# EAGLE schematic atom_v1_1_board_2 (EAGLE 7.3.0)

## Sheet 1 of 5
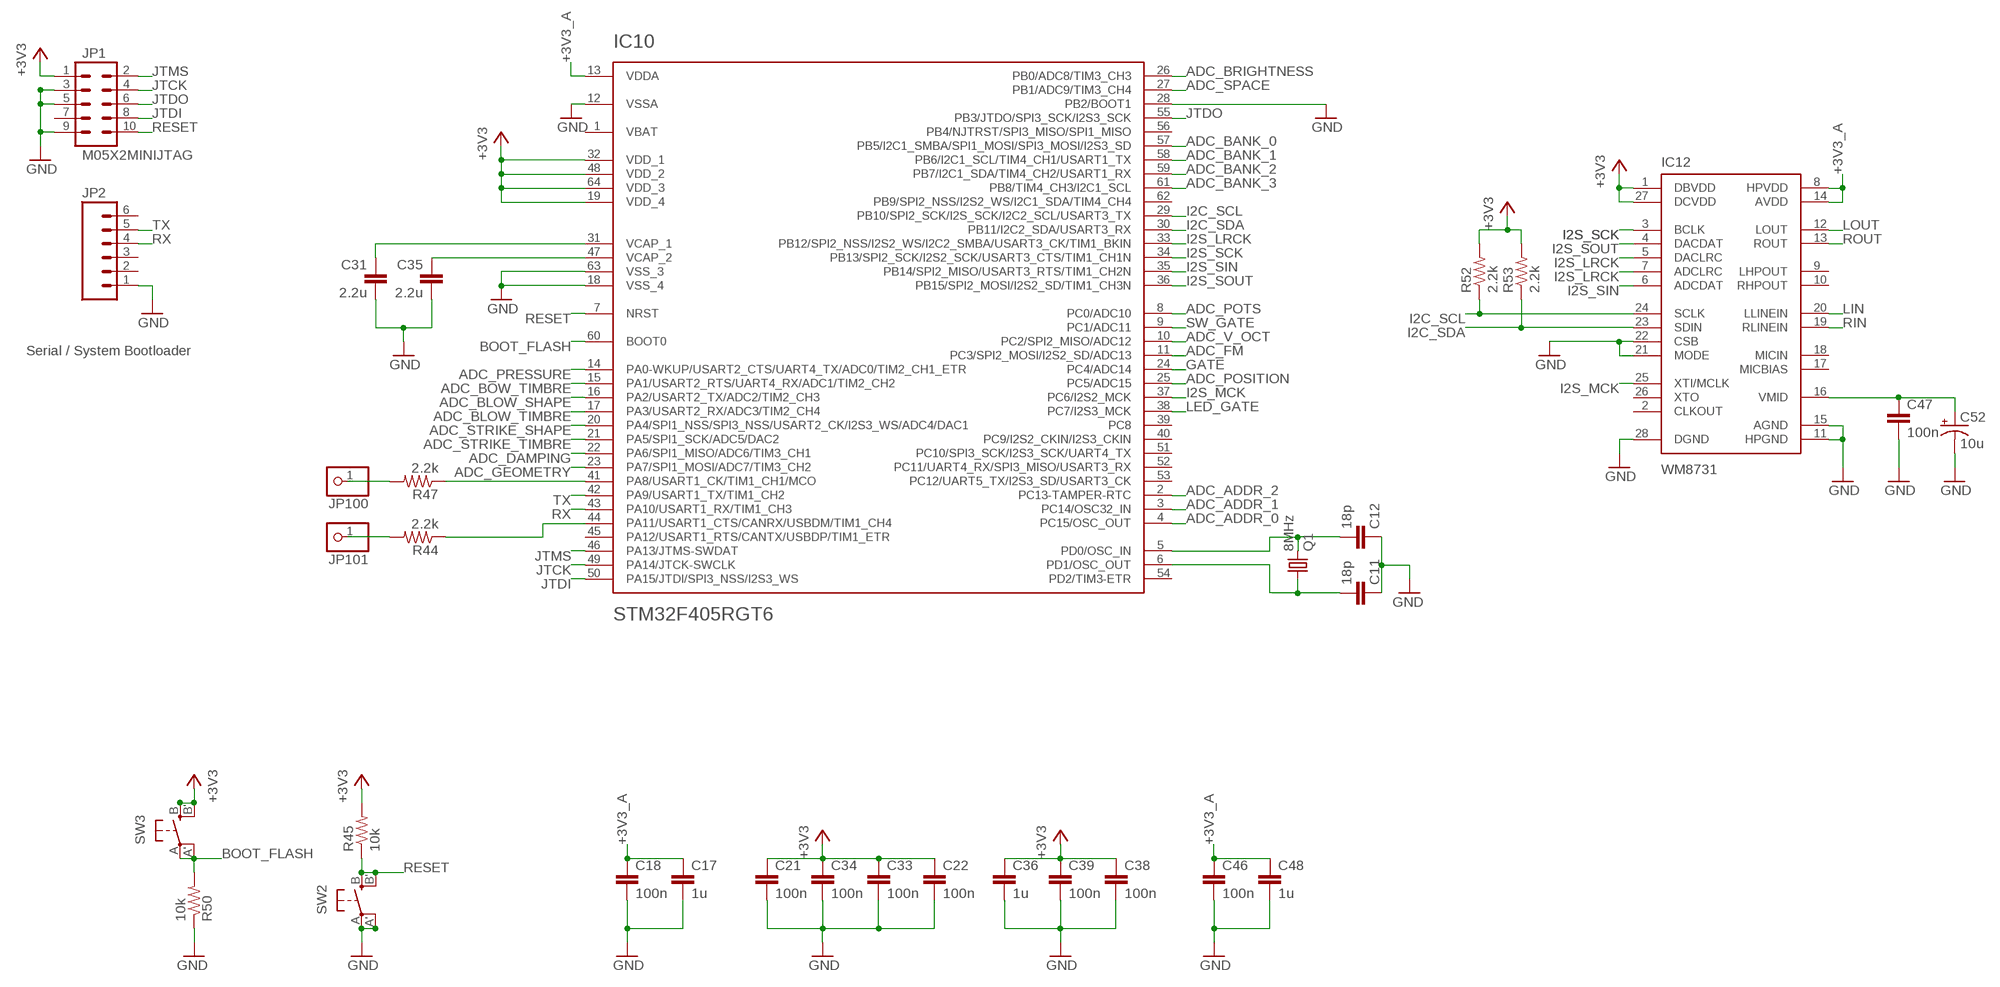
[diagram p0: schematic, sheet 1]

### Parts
C11  18p  CAPACITOR  [RESISTOR_0603]
C12  18p  CAPACITOR  [RESISTOR_0603]
C17  1u  CAPACITOR  [RESISTOR_0603]
C18  100n  CAPACITOR  [RESISTOR_0603]
C21  100n  CAPACITOR  [RESISTOR_0603]
C22  100n  CAPACITOR  [RESISTOR_0603]
C31  2.2u  CAPACITOR  [RESISTOR_0603]
C33  100n  CAPACITOR  [RESISTOR_0603]
C34  100n  CAPACITOR  [RESISTOR_0603]
C35  2.2u  CAPACITOR  [RESISTOR_0603]
C36  1u  CAPACITOR  [RESISTOR_0603]
C38  100n  CAPACITOR  [RESISTOR_0603]
C39  100n  CAPACITOR  [RESISTOR_0603]
C46  100n  CAPACITOR  [RESISTOR_0603]
C47  100n  CAPACITOR  [RESISTOR_0603]
C48  1u  CAPACITOR  [RESISTOR_0603]
C52  10u  CAP_POL  [PANASONIC_B]
IC10  STM32F405RGT6  STM32F20X  [TQFP-10X10-64]
IC12  WM8731  [SSOP28]
JP1  M05X2MINIJTAG  [2X5-1.27]
JP2  M06SIP  [1X06]
JP100  PINHD-1X1  [1X01]
JP101  PINHD-1X1  [1X01]
Q1  8MHz  CRYSTAL  [HC49UP]
R44  2.2k  RESISTOR  [RESISTOR_0603]
R45  10k  RESISTOR  [RESISTOR_0603]
R47  2.2k  RESISTOR  [RESISTOR_0603]
R50  10k  RESISTOR  [RESISTOR_0603]
R52  2.2k  RESISTOR  [RESISTOR_0603]
R53  2.2k  RESISTOR  [RESISTOR_0603]
SW2  EVQQ2  [EVQ-Q2]
SW3  EVQQ2  [EVQ-Q2]

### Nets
+3V3: C21.1 C22.1 C33.1 C34.1 C36.1 C38.1 C39.1 IC10.19(VDD_4) IC10.32(VDD_1) IC10.48(VDD_2) IC10.64(VDD_3) IC12.1(DBVDD) IC12.27(DCVDD) JP1.1 R45.2 R52.2 R53.2 SW3.B'(S1) SW3.B(S) ; also sheet 5
+3V3_A: C17.1 C18.1 C46.1 C48.1 IC10.13(VDDA) IC12.8(HPVDD) IC12.14(AVDD) ; also sheet 3,4,5
ADC_ADDR_0: IC10.4(PC15/OSC_OUT) ; also sheet 4
ADC_ADDR_1: IC10.3(PC14/OSC32_IN) ; also sheet 4
ADC_ADDR_2: IC10.2(PC13-TAMPER-RTC) ; also sheet 4
ADC_BANK_0: IC10.57(PB5/I2C1_SMBA/SPI1_MOSI/SPI3_MOSI/I2S3_SD) ; also sheet 4
ADC_BANK_1: IC10.58(PB6/I2C1_SCL/TIM4_CH1/USART1_TX) ; also sheet 4
ADC_BANK_2: IC10.59(PB7/I2C1_SDA/TIM4_CH2/USART1_RX) ; also sheet 4
ADC_BANK_3: IC10.61(PB8/TIM4_CH3/I2C1_SCL) ; also sheet 4
ADC_BLOW_SHAPE: IC10.16(PA2/USART2_TX/ADC2/TIM2_CH3) ; also sheet 3
ADC_BLOW_TIMBRE: IC10.17(PA3/USART2_RX/ADC3/TIM2_CH4) ; also sheet 3
ADC_BOW_TIMBRE: IC10.15(PA1/USART2_RTS/UART4_RX/ADC1/TIM2_CH2) ; also sheet 3
ADC_BRIGHTNESS: IC10.26(PB0/ADC8/TIM3_CH3) ; also sheet 3
ADC_DAMPING: IC10.22(PA6/SPI1_MISO/ADC6/TIM3_CH1) ; also sheet 3
ADC_FM: IC10.11(PC3/SPI2_MOSI/I2S2_SD/ADC13) ; also sheet 3
ADC_GEOMETRY: IC10.23(PA7/SPI1_MOSI/ADC7/TIM3_CH2) ; also sheet 3
ADC_POSITION: IC10.25(PC5/ADC15) ; also sheet 3
ADC_POTS: IC10.8(PC0/ADC10) ; also sheet 4
ADC_PRESSURE: IC10.14(PA0-WKUP/USART2_CTS/UART4_TX/ADC0/TIM2_CH1_ETR) ; also sheet 3
ADC_SPACE: IC10.27(PB1/ADC9/TIM3_CH4) ; also sheet 3
ADC_STRIKE_SHAPE: IC10.20(PA4/SPI1_NSS/SPI3_NSS/USART2_CK/I2S3_WS/ADC4/DAC1) ; also sheet 3
ADC_STRIKE_TIMBRE: IC10.21(PA5/SPI1_SCK/ADC5/DAC2) ; also sheet 3
ADC_V_OCT: IC10.10(PC2/SPI2_MISO/ADC12) ; also sheet 3
BOOT_FLASH: IC10.60(BOOT0) R50.2 SW3.A'(P1) SW3.A(P)
GATE: IC10.24(PC4/ADC14) ; also sheet 4
GND: C11.1 C12.1 C17.2 C18.2 C21.2 C22.2 C31.2 C33.2 C34.2 C35.2 C36.2 C38.2 C39.2 C46.2 C47.2 C48.2 C52.- IC10.12(VSSA) IC10.18(VSS_4) IC10.28(PB2/BOOT1) IC10.63(VSS_3) IC12.11(HPGND) IC12.15(AGND) IC12.21(MODE) IC12.22(CSB) IC12.28(DGND) JP1.3 JP1.5 JP1.9 JP2.1 R50.1 SW2.A'(P1) SW2.A(P) ; also sheet 2,3,4,5
I2C_SCL: IC10.29(PB10/SPI2_SCK/I2S_SCK/I2C2_SCL/USART3_TX) IC12.24(SCLK) R52.1
I2C_SDA: IC10.30(PB11/I2C2_SDA/USART3_RX) IC12.23(SDIN) R53.1
I2S_LRCK: IC10.33(PB12/SPI2_NSS/I2S2_WS/I2C2_SMBA/USART3_CK/TIM1_BKIN) IC12.5(DACLRC) IC12.7(ADCLRC)
I2S_MCK: IC10.37(PC6/I2S2_MCK) IC12.25(XTI/MCLK)
I2S_SCK: IC10.34(PB13/SPI2_SCK/I2S2_SCK/USART3_CTS/TIM1_CH1N) IC12.3(BCLK)
I2S_SIN: IC10.35(PB14/SPI2_MISO/USART3_RTS/TIM1_CH2N) IC12.6(ADCDAT)
I2S_SOUT: IC10.36(PB15/SPI2_MOSI/I2S2_SD/TIM1_CH3N) IC12.4(DACDAT)
JTCK: IC10.49(PA14/JTCK-SWCLK) JP1.4
JTDI: IC10.50(PA15/JTDI/SPI3_NSS/I2S3_WS) JP1.8
JTDO: IC10.55(PB3/JTDO/SPI3_SCK/I2S3_SCK) JP1.6
JTMS: IC10.46(PA13/JTMS-SWDAT) JP1.2
LED_GATE: IC10.38(PC7/I2S3_MCK) ; also sheet 4
LIN: IC12.20(LLINEIN) ; also sheet 2
LOUT: IC12.12(LOUT) ; also sheet 2
N$7: C12.2 IC10.5(PD0/OSC_IN) Q1.2
N$8: C11.2 IC10.6(PD1/OSC_OUT) Q1.1
N$13: C35.1 IC10.47(VCAP_2)
N$17: C47.1 C52.+ IC12.16(VMID)
N$19: C31.1 IC10.31(VCAP_1)
N$54: IC10.44(PA11/USART1_CTS/CANRX/USBDM/TIM1_CH4) R44.1
N$79: IC10.41(PA8/USART1_CK/TIM1_CH1/MCO) R47.1
N$129: JP100.1 R47.2
N$130: JP101.1 R44.2
RESET: IC10.7(NRST) JP1.10 R45.1 SW2.B'(S1) SW2.B(S)
RIN: IC12.19(RLINEIN) ; also sheet 2
ROUT: IC12.13(ROUT) ; also sheet 2
RX: IC10.43(PA10/USART1_RX/TIM1_CH3) JP2.4
SW_GATE: IC10.9(PC1/ADC11) ; also sheet 4
TX: IC10.42(PA9/USART1_TX/TIM1_CH2) JP2.5
Unconnected: IC10.39(PC8) IC10.40(PC9/I2S2_CKIN/I2S3_CKIN) IC10.45(PA12/USART1_RTS/CANTX/USBDP/TIM1_ETR) IC10.51(PC10/SPI3_SCK/I2S3_SCK/UART4_TX) IC10.52(PC11/UART4_RX/SPI3_MISO/USART3_RX) IC10.53(PC12/UART5_TX/I2S3_SD/USART3_CK) IC10.54(PD2/TIM3-ETR) IC10.56(PB4/NJTRST/SPI3_MISO/SPI1_MISO) IC10.62(PB9/SPI2_NSS/I2S2_WS/I2C1_SDA/TIM4_CH4) IC12.2(CLKOUT) IC12.9(LHPOUT) IC12.10(RHPOUT) IC12.17(MICBIAS) IC12.18(MICIN) IC12.26(XTO) JP1.7 JP2.2 JP2.3 JP2.6

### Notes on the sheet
- Serial / System Bootloader

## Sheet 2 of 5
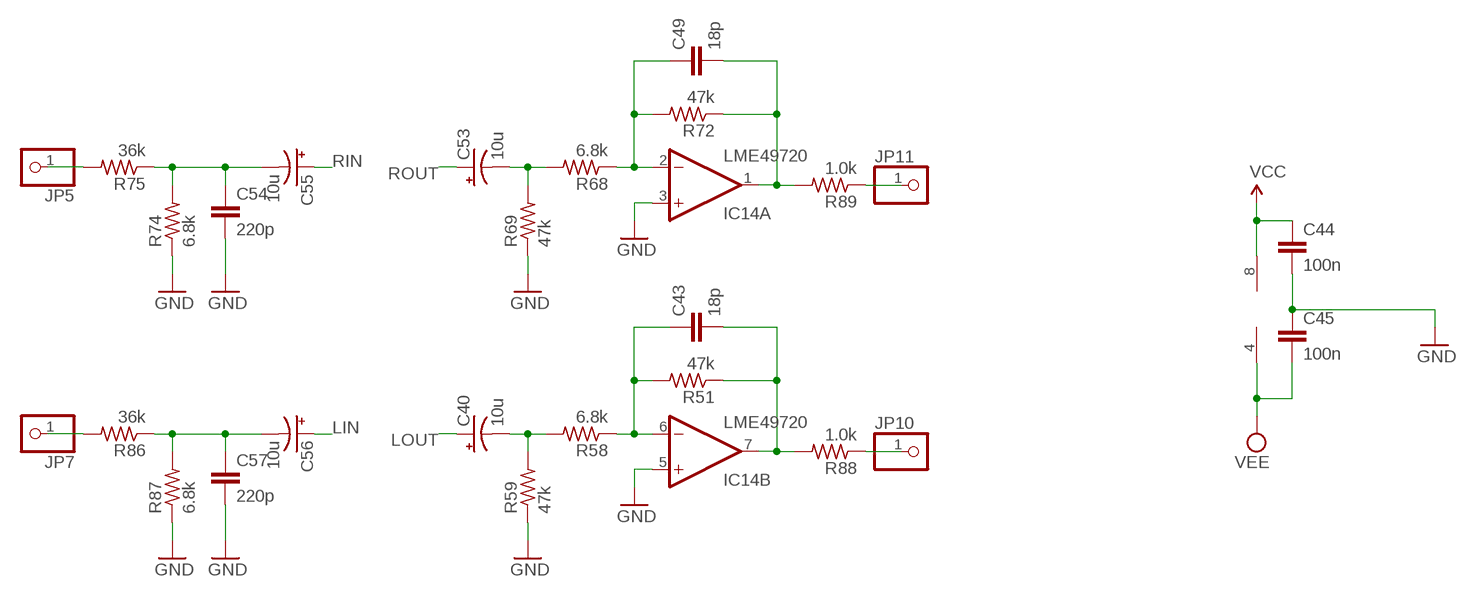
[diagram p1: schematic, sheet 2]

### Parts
C40  10u  CAP_POL  [PANASONIC_B]
C43  18p  CAPACITOR  [RESISTOR_0603]
C44  100n  CAPACITOR  [RESISTOR_0603]
C45  100n  CAPACITOR  [RESISTOR_0603]
C49  18p  CAPACITOR  [RESISTOR_0603]
C53  10u  CAP_POL  [PANASONIC_B]
C54  220p  CAPACITOR  [RESISTOR_0603]
C55  10u  CAP_POL  [PANASONIC_B]
C56  10u  CAP_POL  [PANASONIC_B]
C57  220p  CAPACITOR  [RESISTOR_0603]
IC14  LME49720  TL072D  [SO08]
JP5  PINHD-1X1  [1X01]
JP7  PINHD-1X1  [1X01]
JP10  PINHD-1X1  [1X01]
JP11  PINHD-1X1  [1X01]
R51  47k  RESISTOR  [RESISTOR_0603]
R58  6.8k  RESISTOR  [RESISTOR_0603]
R59  47k  RESISTOR  [RESISTOR_0603]
R68  6.8k  RESISTOR  [RESISTOR_0603]
R69  47k  RESISTOR  [RESISTOR_0603]
R72  47k  RESISTOR  [RESISTOR_0603]
R74  6.8k  RESISTOR  [RESISTOR_0603]
R75  36k  RESISTOR  [RESISTOR_0603]
R86  36k  RESISTOR  [RESISTOR_0603]
R87  6.8k  RESISTOR  [RESISTOR_0603]
R88  1.0k  RESISTOR  [RESISTOR_0603]
R89  1.0k  RESISTOR  [RESISTOR_0603]

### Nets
GND: C44.2 C45.1 C54.2 C57.2 IC14.3(A:+IN) IC14.5(B:+IN) R59.1 R69.1 R74.1 R87.1 ; also sheet 1,3,4,5
LIN: C56.+ ; also sheet 1
LOUT: C40.+ ; also sheet 1
N$18: C56.- C57.1 R86.1 R87.2
N$22: C54.1 C55.- R74.2 R75.1
N$23: C40.- R58.2 R59.2
N$25: C43.1 IC14.6(B:-IN) R51.2 R58.1
N$28: C43.2 IC14.7(B:OUT) R51.1 R88.2
N$31: C53.- R68.2 R69.2
N$32: C49.1 IC14.2(A:-IN) R68.1 R72.2
N$33: C49.2 IC14.1(A:OUT) R72.1 R89.2
N$81: JP5.1 R75.2
N$82: JP11.1 R89.1
N$84: JP10.1 R88.1
N$86: JP7.1 R86.2
RIN: C55.+ ; also sheet 1
ROUT: C53.+ ; also sheet 1
VCC [wide]: C44.1 IC14.8(P:V+) ; also sheet 5
VEE [wide]: C45.2 IC14.4(P:V-) ; also sheet 5

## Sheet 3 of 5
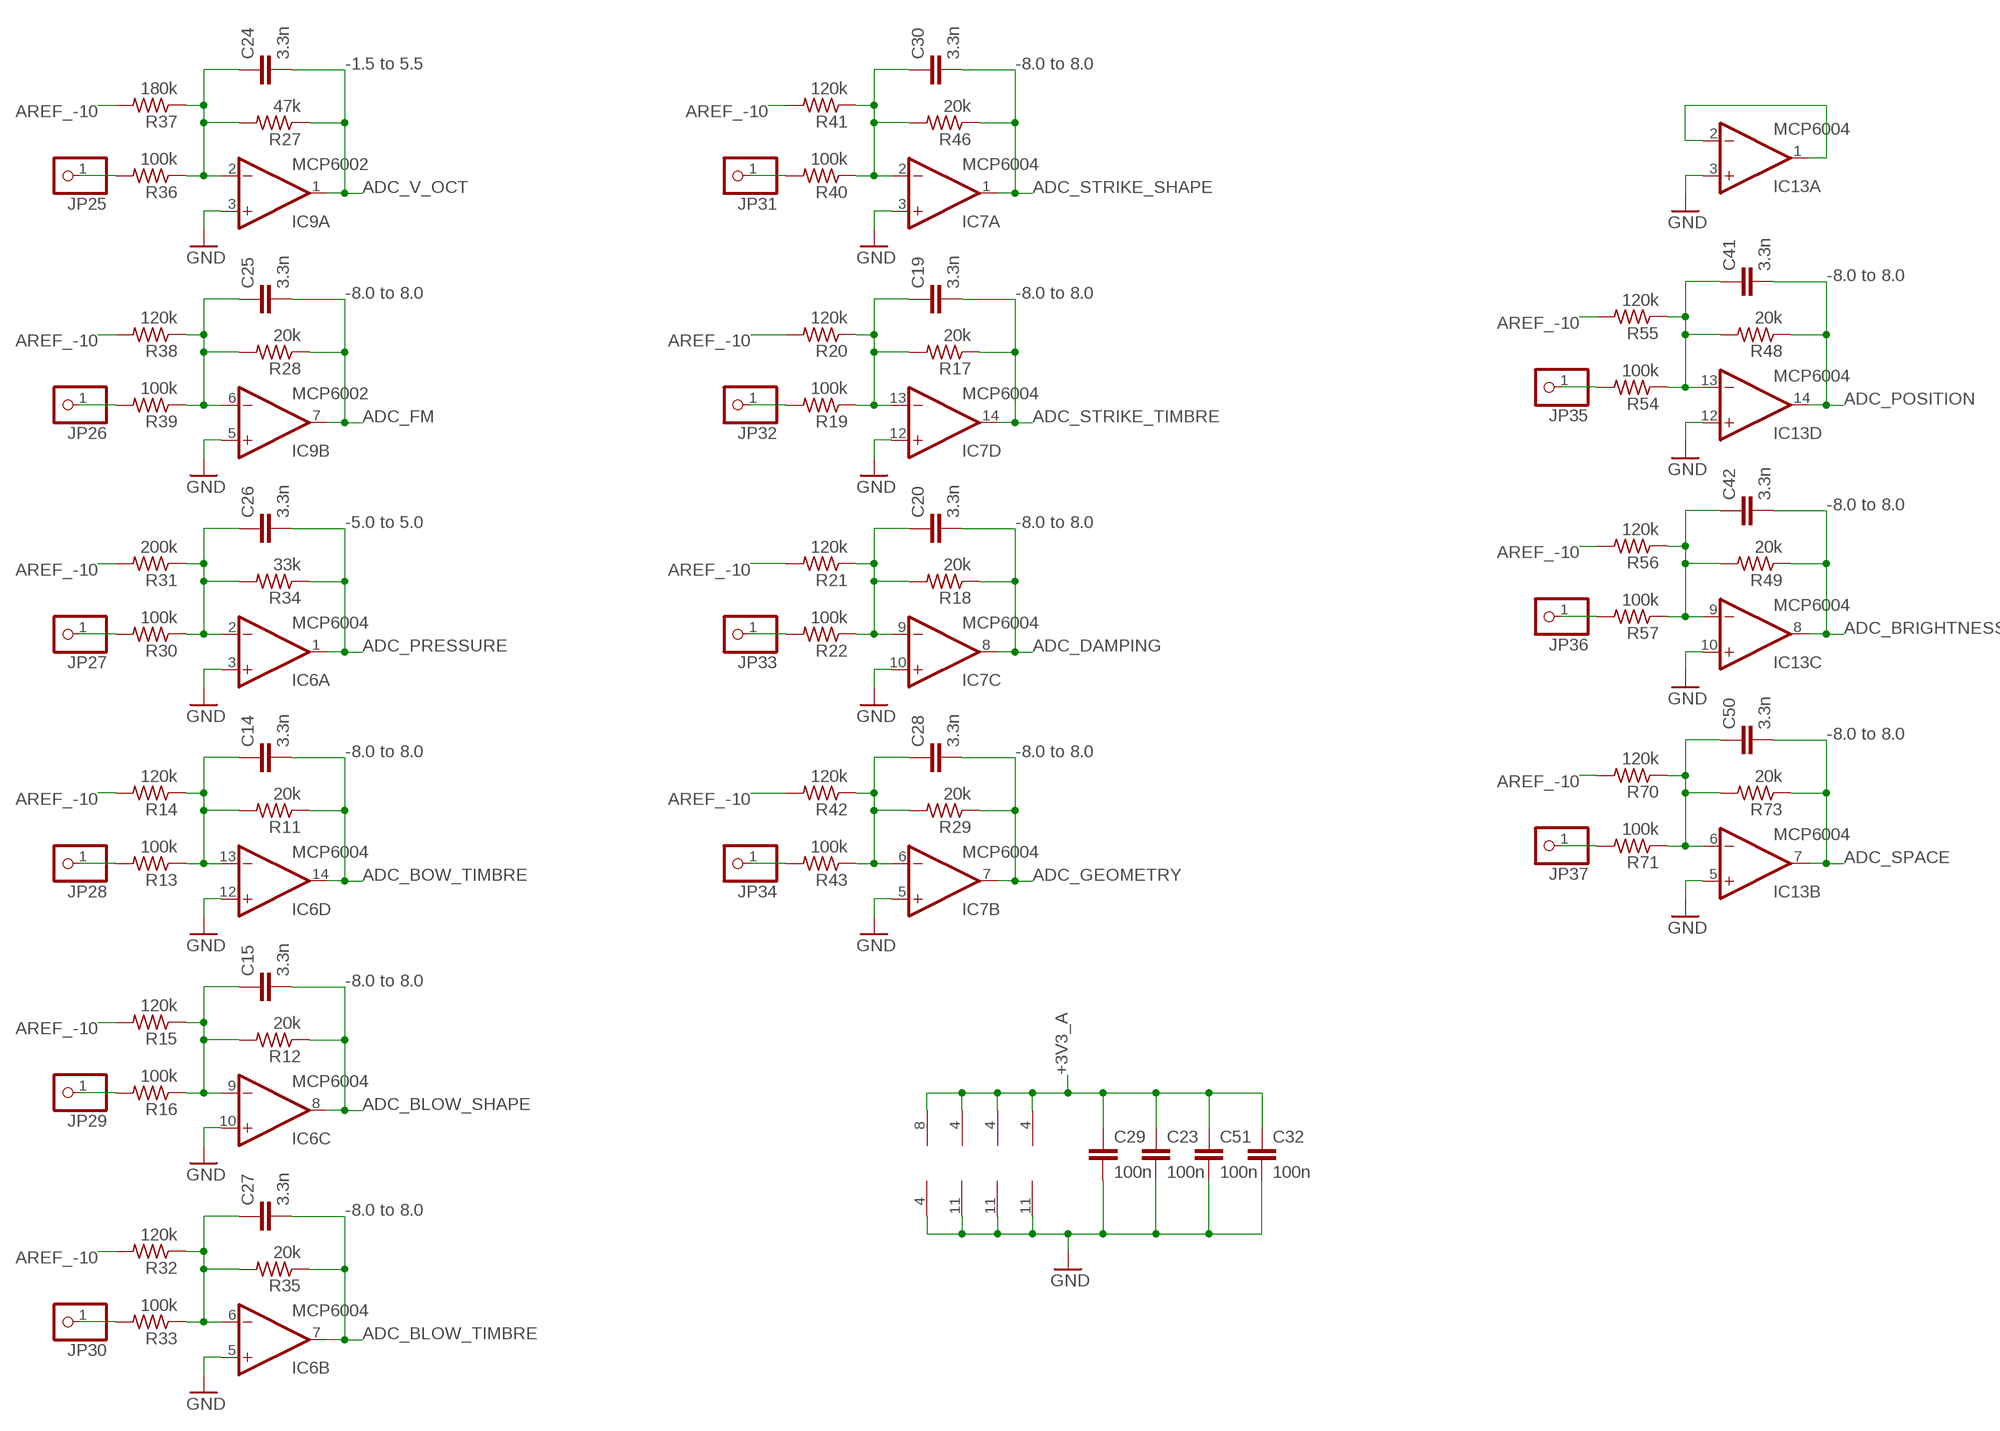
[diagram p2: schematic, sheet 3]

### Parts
C14  3.3n  CAPACITOR  [RESISTOR_0603]
C15  3.3n  CAPACITOR  [RESISTOR_0603]
C19  3.3n  CAPACITOR  [RESISTOR_0603]
C20  3.3n  CAPACITOR  [RESISTOR_0603]
C23  100n  CAPACITOR  [RESISTOR_0603]
C24  3.3n  CAPACITOR  [RESISTOR_0603]
C25  3.3n  CAPACITOR  [RESISTOR_0603]
C26  3.3n  CAPACITOR  [RESISTOR_0603]
C27  3.3n  CAPACITOR  [RESISTOR_0603]
C28  3.3n  CAPACITOR  [RESISTOR_0603]
C29  100n  CAPACITOR  [RESISTOR_0603]
C30  3.3n  CAPACITOR  [RESISTOR_0603]
C32  100n  CAPACITOR  [RESISTOR_0603]
C41  3.3n  CAPACITOR  [RESISTOR_0603]
C42  3.3n  CAPACITOR  [RESISTOR_0603]
C50  3.3n  CAPACITOR  [RESISTOR_0603]
C51  100n  CAPACITOR  [RESISTOR_0603]
IC6  MCP6004  TL074D  [SO14]
IC7  MCP6004  TL074D  [SO14]
IC9  MCP6002  TL072D  [SO08]
IC13  MCP6004  TL074D  [SO14]
JP25  PINHD-1X1  [1X01]
JP26  PINHD-1X1  [1X01]
JP27  PINHD-1X1  [1X01]
JP28  PINHD-1X1  [1X01]
JP29  PINHD-1X1  [1X01]
JP30  PINHD-1X1  [1X01]
JP31  PINHD-1X1  [1X01]
JP32  PINHD-1X1  [1X01]
JP33  PINHD-1X1  [1X01]
JP34  PINHD-1X1  [1X01]
JP35  PINHD-1X1  [1X01]
JP36  PINHD-1X1  [1X01]
JP37  PINHD-1X1  [1X01]
R11  20k  RESISTOR  [RESISTOR_0603]
R12  20k  RESISTOR  [RESISTOR_0603]
R13  100k  RESISTOR  [RESISTOR_0603]
R14  120k  RESISTOR  [RESISTOR_0603]
R15  120k  RESISTOR  [RESISTOR_0603]
R16  100k  RESISTOR  [RESISTOR_0603]
R17  20k  RESISTOR  [RESISTOR_0603]
R18  20k  RESISTOR  [RESISTOR_0603]
R19  100k  RESISTOR  [RESISTOR_0603]
R20  120k  RESISTOR  [RESISTOR_0603]
R21  120k  RESISTOR  [RESISTOR_0603]
R22  100k  RESISTOR  [RESISTOR_0603]
R27  47k  RESISTOR  [RESISTOR_0603]
R28  20k  RESISTOR  [RESISTOR_0603]
R29  20k  RESISTOR  [RESISTOR_0603]
R30  100k  RESISTOR  [RESISTOR_0603]
R31  200k  RESISTOR  [RESISTOR_0603]
R32  120k  RESISTOR  [RESISTOR_0603]
R33  100k  RESISTOR  [RESISTOR_0603]
R34  33k  RESISTOR  [RESISTOR_0603]
R35  20k  RESISTOR  [RESISTOR_0603]
R36  100k  RESISTOR  [RESISTOR_0603]
R37  180k  RESISTOR  [RESISTOR_0603]
R38  120k  RESISTOR  [RESISTOR_0603]
R39  100k  RESISTOR  [RESISTOR_0603]
R40  100k  RESISTOR  [RESISTOR_0603]
R41  120k  RESISTOR  [RESISTOR_0603]
R42  120k  RESISTOR  [RESISTOR_0603]
R43  100k  RESISTOR  [RESISTOR_0603]
R46  20k  RESISTOR  [RESISTOR_0603]
R48  20k  RESISTOR  [RESISTOR_0603]
R49  20k  RESISTOR  [RESISTOR_0603]
R54  100k  RESISTOR  [RESISTOR_0603]
R55  120k  RESISTOR  [RESISTOR_0603]
R56  120k  RESISTOR  [RESISTOR_0603]
R57  100k  RESISTOR  [RESISTOR_0603]
R70  120k  RESISTOR  [RESISTOR_0603]
R71  100k  RESISTOR  [RESISTOR_0603]
R73  20k  RESISTOR  [RESISTOR_0603]

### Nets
+3V3_A: C23.1 C29.1 C32.1 C51.1 IC6.4(P:V+) IC7.4(P:V+) IC9.8(P:V+) IC13.4(P:V+) ; also sheet 1,4,5
ADC_BLOW_SHAPE: C15.2 IC6.8(C:OUT) R12.1 ; also sheet 1
ADC_BLOW_TIMBRE: C27.2 IC6.7(B:OUT) R35.1 ; also sheet 1
ADC_BOW_TIMBRE: C14.2 IC6.14(D:OUT) R11.1 ; also sheet 1
ADC_BRIGHTNESS: C42.2 IC13.8(C:OUT) R49.1 ; also sheet 1
ADC_DAMPING: C20.2 IC7.8(C:OUT) R18.1 ; also sheet 1
ADC_FM: C25.2 IC9.7(B:OUT) R28.1 ; also sheet 1
ADC_GEOMETRY: C28.2 IC7.7(B:OUT) R29.1 ; also sheet 1
ADC_POSITION: C41.2 IC13.14(D:OUT) R48.1 ; also sheet 1
ADC_PRESSURE: C26.2 IC6.1(A:OUT) R34.1 ; also sheet 1
ADC_SPACE: C50.2 IC13.7(B:OUT) R73.1 ; also sheet 1
ADC_STRIKE_SHAPE: C30.2 IC7.1(A:OUT) R46.1 ; also sheet 1
ADC_STRIKE_TIMBRE: C19.2 IC7.14(D:OUT) R17.1 ; also sheet 1
ADC_V_OCT: C24.2 IC9.1(A:OUT) R27.1 ; also sheet 1
AREF_-10: R14.2 R15.2 R20.2 R21.2 R31.2 R32.2 R37.2 R38.2 R41.2 R42.2 R55.2 R56.2 R70.2 ; also sheet 5
GND: C23.2 C29.2 C32.2 C51.2 IC6.3(A:+IN) IC6.5(B:+IN) IC6.10(C:+IN) IC6.11(P:V-) IC6.12(D:+IN) IC7.3(A:+IN) IC7.5(B:+IN) IC7.10(C:+IN) IC7.11(P:V-) IC7.12(D:+IN) IC9.3(A:+IN) IC9.4(P:V-) IC9.5(B:+IN) IC13.3(A:+IN) IC13.5(B:+IN) IC13.10(C:+IN) IC13.11(P:V-) IC13.12(D:+IN) ; also sheet 1,2,4,5
N$2: C15.1 IC6.9(C:-IN) R12.2 R15.1 R16.1
N$4: JP25.1 R36.2
N$5: C14.1 IC6.13(D:-IN) R11.2 R13.1 R14.1
N$9: C19.1 IC7.13(D:-IN) R17.2 R19.1 R20.1
N$10: JP26.1 R39.2
N$11: C24.1 IC9.2(A:-IN) R27.2 R36.1 R37.1
N$14: C20.1 IC7.9(C:-IN) R18.2 R21.1 R22.1
N$15: C25.1 IC9.6(B:-IN) R28.2 R38.1 R39.1
N$24: C30.1 IC7.2(A:-IN) R40.1 R41.1 R46.2
N$27: C27.1 IC6.6(B:-IN) R32.1 R33.1 R35.2
N$30: C42.1 IC13.9(C:-IN) R49.2 R56.1 R57.1
N$35: C50.1 IC13.6(B:-IN) R70.1 R71.1 R73.2
N$37: C28.1 IC7.6(B:-IN) R29.2 R42.1 R43.1
N$40: C41.1 IC13.13(D:-IN) R48.2 R54.1 R55.1
N$41: JP27.1 R30.2
N$42: C26.1 IC6.2(A:-IN) R30.1 R31.1 R34.2
N$44: IC13.1(A:OUT) IC13.2(A:-IN)
N$87: JP28.1 R13.2
N$88: JP29.1 R16.2
N$89: JP30.1 R33.2
N$93: JP31.1 R40.2
N$94: JP32.1 R19.2
N$95: JP33.1 R22.2
N$96: JP34.1 R43.2
N$97: JP37.1 R71.2
N$98: JP36.1 R57.2
N$99: JP35.1 R54.2

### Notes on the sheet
- -1.5 to 5.5 | -8.0 to 8.0
- -8.0 to 8.0
- -8.0 to 8.0 | -8.0 to 8.0
- -8.0 to 8.0
- -5.0 to 5.0 | -8.0 to 8.0
- -8.0 to 8.0
- -8.0 to 8.0 | -8.0 to 8.0
- -8.0 to 8.0
- -8.0 to 8.0

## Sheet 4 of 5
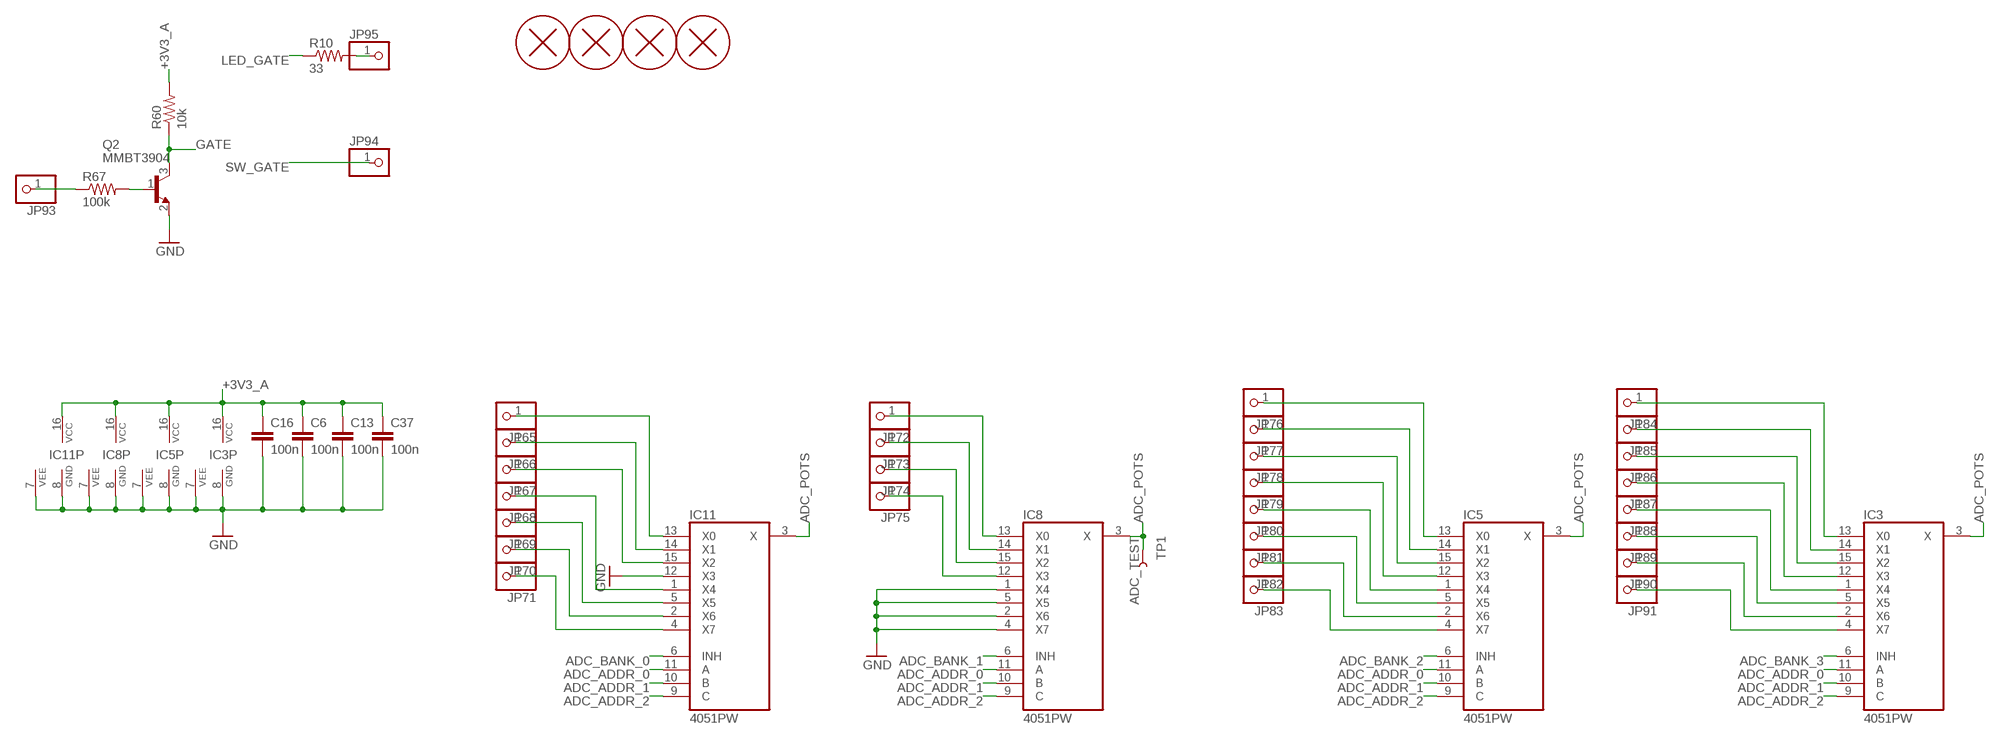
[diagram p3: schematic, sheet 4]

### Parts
C6  100n  CAPACITOR  [RESISTOR_0603]
C13  100n  CAPACITOR  [RESISTOR_0603]
C16  100n  CAPACITOR  [RESISTOR_0603]
C37  100n  CAPACITOR  [RESISTOR_0603]
H1  PCB_SCREW  [PCB_SCREW]
H2  PCB_SCREW  [PCB_SCREW]
H3  PCB_SCREW  [PCB_SCREW]
H4  PCB_SCREW  [PCB_SCREW]
IC3  4051PW  [TSSOP16]
IC5  4051PW  [TSSOP16]
IC8  4051PW  [TSSOP16]
IC11  4051PW  [TSSOP16]
JP65  PINHD-1X1  [1X01]
JP66  PINHD-1X1  [1X01]
JP67  PINHD-1X1  [1X01]
JP68  PINHD-1X1  [1X01]
JP69  PINHD-1X1  [1X01]
JP70  PINHD-1X1  [1X01]
JP71  PINHD-1X1  [1X01]
JP72  PINHD-1X1  [1X01]
JP73  PINHD-1X1  [1X01]
JP74  PINHD-1X1  [1X01]
JP75  PINHD-1X1  [1X01]
JP76  PINHD-1X1  [1X01]
JP77  PINHD-1X1  [1X01]
JP78  PINHD-1X1  [1X01]
JP79  PINHD-1X1  [1X01]
JP80  PINHD-1X1  [1X01]
JP81  PINHD-1X1  [1X01]
JP82  PINHD-1X1  [1X01]
JP83  PINHD-1X1  [1X01]
JP84  PINHD-1X1  [1X01]
JP85  PINHD-1X1  [1X01]
JP86  PINHD-1X1  [1X01]
JP87  PINHD-1X1  [1X01]
JP88  PINHD-1X1  [1X01]
JP89  PINHD-1X1  [1X01]
JP90  PINHD-1X1  [1X01]
JP91  PINHD-1X1  [1X01]
JP93  PINHD-1X1  [1X01]
JP94  PINHD-1X1  [1X01]
JP95  PINHD-1X1  [1X01]
Q2  MMBT3904  MMBT3904SOT23  [SOT23]
R10  33  RESISTOR  [RESISTOR_0603]
R60  10k  RESISTOR  [RESISTOR_0603]
R67  100k  RESISTOR  [RESISTOR_0603]
TP1  ADC_TEST  TEST-POINT3  [PAD.03X.03]

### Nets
+3V3_A: C6.1 C13.1 C16.1 C37.1 IC3.16(VCC) IC5.16(VCC) IC8.16(VCC) IC11.16(VCC) R60.2 ; also sheet 1,3,5
ADC_ADDR_0: IC3.11(A) IC5.11(A) IC8.11(A) IC11.11(A) ; also sheet 1
ADC_ADDR_1: IC3.10(B) IC5.10(B) IC8.10(B) IC11.10(B) ; also sheet 1
ADC_ADDR_2: IC3.9(C) IC5.9(C) IC8.9(C) IC11.9(C) ; also sheet 1
ADC_BANK_0: IC11.6(INH) ; also sheet 1
ADC_BANK_1: IC8.6(INH) ; also sheet 1
ADC_BANK_2: IC5.6(INH) ; also sheet 1
ADC_BANK_3: IC3.6(INH) ; also sheet 1
ADC_POTS: IC3.3(X) IC5.3(X) IC8.3(X) IC11.3(X) TP1.P$1 ; also sheet 1
GATE: Q2.3(C) R60.1 ; also sheet 1
GND: C6.2 C13.2 C16.2 C37.2 IC3.7(VEE) IC3.8(GND) IC5.7(VEE) IC5.8(GND) IC8.1(X4) IC8.2(X6) IC8.4(X7) IC8.5(X5) IC8.7(VEE) IC8.8(GND) IC11.7(VEE) IC11.8(GND) IC11.12(X3) Q2.2(E) ; also sheet 1,2,3,5
LED_GATE: R10.1 ; also sheet 1
N$38: JP95.1 R10.2
N$66: Q2.1(B) R67.2
N$100: IC11.13(X0) JP65.1
N$101: IC11.14(X1) JP66.1
N$102: IC11.15(X2) JP67.1
N$103: IC11.1(X4) JP68.1
N$104: IC11.5(X5) JP69.1
N$105: IC11.2(X6) JP70.1
N$106: IC11.4(X7) JP71.1
N$107: IC8.13(X0) JP72.1
N$108: IC8.14(X1) JP73.1
N$109: IC8.15(X2) JP74.1
N$110: IC8.12(X3) JP75.1
N$111: IC5.13(X0) JP76.1
N$112: IC5.14(X1) JP77.1
N$113: IC5.15(X2) JP78.1
N$114: IC5.12(X3) JP79.1
N$115: IC5.1(X4) JP80.1
N$116: IC5.5(X5) JP81.1
N$117: IC5.2(X6) JP82.1
N$118: IC5.4(X7) JP83.1
N$119: IC3.13(X0) JP84.1
N$120: IC3.14(X1) JP85.1
N$121: IC3.15(X2) JP86.1
N$122: IC3.12(X3) JP87.1
N$123: IC3.1(X4) JP88.1
N$124: IC3.5(X5) JP89.1
N$125: IC3.2(X6) JP90.1
N$126: IC3.4(X7) JP91.1
N$127: JP93.1 R67.1
SW_GATE: JP94.1 ; also sheet 1

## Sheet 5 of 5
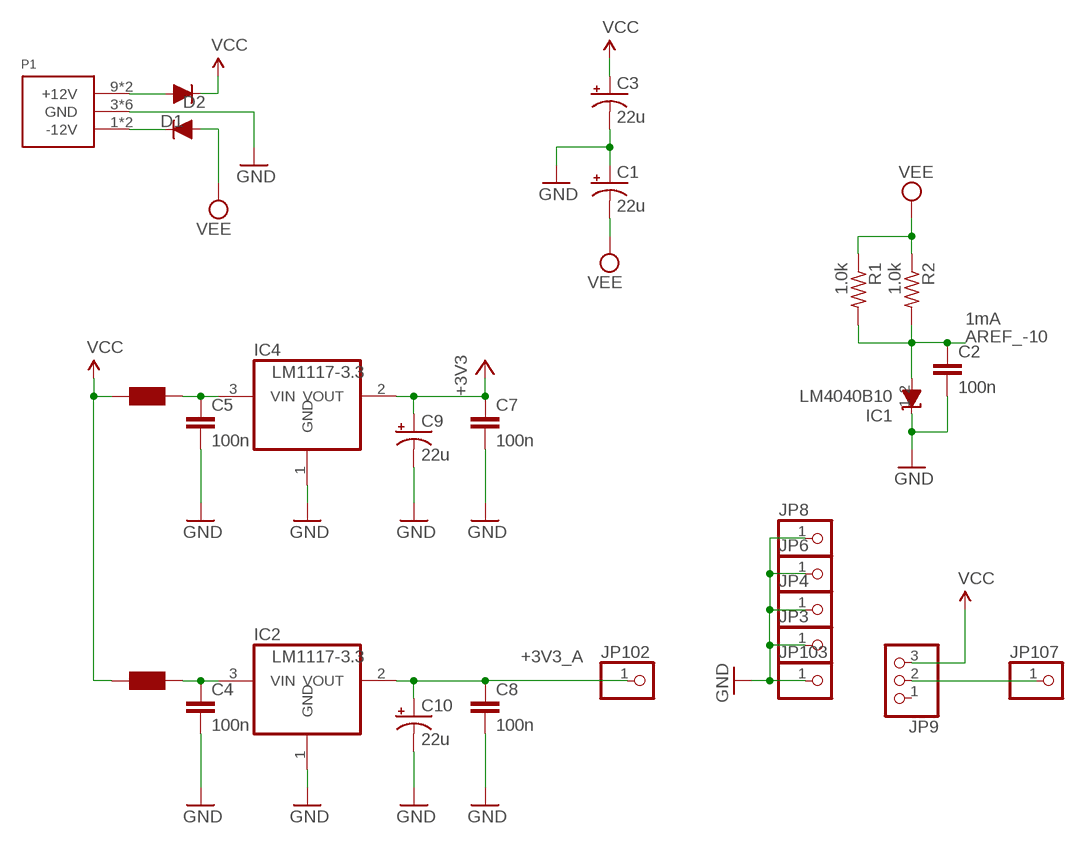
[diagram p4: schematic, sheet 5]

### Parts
C1  22u  CAP_POLD  [PANASONIC_D]
C2  100n  CAPACITOR  [RESISTOR_0603]
C3  22u  CAP_POLD  [PANASONIC_D]
C4  100n  CAPACITOR  [RESISTOR_0603]
C5  100n  CAPACITOR  [RESISTOR_0603]
C7  100n  CAPACITOR  [RESISTOR_0603]
C8  100n  CAPACITOR  [RESISTOR_0603]
C9  22u  CAP_POLD  [PANASONIC_D]
C10  22u  CAP_POLD  [PANASONIC_D]
D1  1N5819HW  DIODE  [SOD123]
D2  1N5819HW  DIODE  [SOD123]
F1  FERRITE-BEAD  [RESISTOR_0603]
F2  FERRITE-BEAD  [RESISTOR_0603]
IC1  LM4040B10  LM4040SOT23  [SOT23]
IC2  LM1117-3.3  REG1117  [SOT223]
IC4  LM1117-3.3  REG1117  [SOT223]
JP3  PINHD-1X1  [1X01]
JP4  PINHD-1X1  [1X01]
JP6  PINHD-1X1  [1X01]
JP8  PINHD-1X1  [1X01]
JP9  PINHD-1X3  [1X03]
JP102  PINHD-1X1  [1X01]
JP103  PINHD-1X1  [1X01]
JP107  PINHD-1X1  [1X01]
P1  POWER_SIMPLE10  [POWER_10]
R1  1.0k  RESISTOR  [RESISTOR_0603]
R2  1.0k  RESISTOR  [RESISTOR_0603]

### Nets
+3V3: C7.1 C9.+ IC4.2(VOUT) ; also sheet 1
+3V3_A: C8.1 C10.+ IC2.2(VOUT) JP102.1 ; also sheet 1,3,4
AREF_-10: C2.1 IC1.2(A) R1.2 R2.2 ; also sheet 3
GND: C1.+ C2.2 C3.- C4.2 C5.2 C7.2 C8.2 C9.- C10.- IC1.1(C) IC2.1(GND) IC4.1(GND) JP3.1 JP4.1 JP6.1 JP8.1 JP103.1 P1.3(GND) P1.4(GND) P1.5(GND) P1.6(GND) P1.7(GND) P1.8(GND) ; also sheet 1,2,3,4
N$1 [wide]: D1.+ P1.9(+12V) P1.10(+12V)
N$3 [wide]: D2.- P1.1(-12V) P1.2(-12V)
N$6 [wide]: JP9.2 JP107.1
N$61 [wide]: C5.1 F1.1 IC4.3(VIN)
N$80 [wide]: C4.1 F2.1 IC2.3(VIN)
VCC [wide]: C3.+ D1.- F1.2 F2.2 JP9.3 ; also sheet 2
VEE [wide]: C1.- D2.+ R1.1 R2.1 ; also sheet 2
Unconnected: JP9.1

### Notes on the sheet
- 1mA

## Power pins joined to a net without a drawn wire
VBAT: IC10.1(VBAT)

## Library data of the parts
C1 C3 C9 C10 C40 C52 C53 C55 C56 = parts_aman:CAP_POL
C2 C4-C8 C11-C39 C41-C51 C54 C57 = parts_aman:CAPACITOR
D1 D2 = parts_aman:DIODE
F1 F2 = parts_aman:FERRITE-BEAD
H1-H4 = parts_aman:PCB_SCREW
IC1 = parts_aman:LM4040
IC2 IC4 = og-vreg:REG1117: 800mA and 1A Low Dropout (LDO) Positive Regulator 1.8V, 2.5V, 2.85V, 3.3V, 5V, and Adj
IC3 IC5 IC8 IC11 = og-ics:4051: 8-channel ANALOG MULTIPLEXER
IC6 IC7 IC13 = gm-ics:TL074: OP AMP
IC9 = gm-ics:TL072: OP AMP
IC10 = og-stm32f2:STM32F20X
IC12 = og-dac:WM8731
IC14 = og-linear:TL072: OP AMP
JP1 = og-header:M05X2: Header 5x2 Standard 10-pin dual row 0.1" header. Commonly used with AVR-ISP. Use with Spark Fun Electronics SKU: PRT-00778
JP2 = SparkFun:M06: Header 6 Standard 6-pin 0.1" header. Use with straight break away headers (SKU : PRT-00116), right angle break away headers (PRT-00553), swiss pins (PRT-00743), machine pins (PRT-00117), and female headers (PRT-00115). Molex polarized connector foot print use with SKU : PRT-08094 with associated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
JP3-JP8 JP10 JP11 JP25-JP37 JP65-JP91 JP93-JP95 JP100-JP103 JP107 = parts_aman:PINHD-1X1: PIN HEADER
JP9 = parts_aman:PINHD-1X3: PIN HEADER
P1 = parts_aman:POWER_SIMPLE
Q1 = parts_aman:CRYSTAL
Q2 = parts_aman:MMBT3904
R1 R2 R10-R22 R27-R60 R67-R75 R86-R89 = parts_aman:RESISTOR
SW2 SW3 = adafruit:EVQQ2: SMT 6mm switch, EVQQ2 series http://www.ladyada.net/library/eagle
TP1 = SparkFun:TEST-POINT

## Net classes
0 default: width 0.152 mm, drill 0.305 mm, clearance 0.152 mm
1 wide: width 0.305 mm, drill 0.305 mm, clearance 0.305 mm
